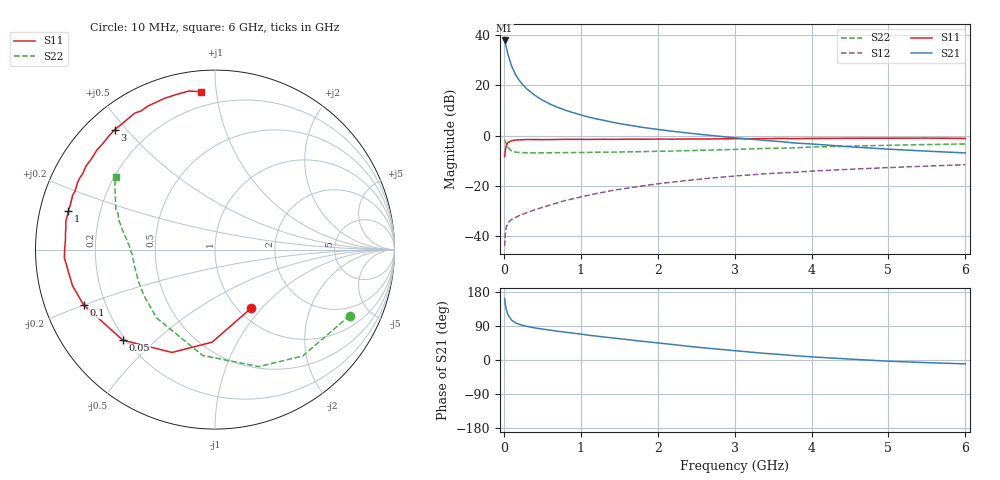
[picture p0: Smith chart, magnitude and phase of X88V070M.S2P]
! SIEMENS Small Signal Semiconductors
! BFP136W
! Si NPN RF Bipolar Junction Transistor in SOT343
! VCE = 8 V  IC = 70 mA
! Common Emitter S-Parameters:  September  1994
# GHz  S  MA  R  50
!  f  S11  S21  S12  S22
! GHz  MAG  ANG  MAG  ANG  MAG  ANG  MAG  ANG
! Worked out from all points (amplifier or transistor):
!   40 points, 10 MHz to 6 GHz, reference 50 ohm
!   highest |S21| = 37.8 dB at 10 MHz (marker M1)
!   |S21| within 3 dB of that: start of sweep to 34.34 MHz
!   unconditionally stable (mu >= 1): 640.7 MHz to 2.969 GHz
!   at 200 MHz: K = 0.58, MSG = 26.9 dB, |S12| = -31.7 dB
!   at 1.5 GHz: K = 1.11, MAG = 11.1 dB, |S12| = -21.3 dB
!   at 6 GHz: K = 0.96, MSG = 2.3 dB, |S12| = -11.5 dB
!   S11 on the Smith chart (normalised r, x): 10 MHz: 1.15, -0.88; 50 MHz: 0.19, -0.40; 100 MHz: 0.12, -0.20; 1 GHz: 0.09, +0.13; 3 GHz: 0.08, +0.46; 6 GHz: 0.11, +0.91
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0.01  0.3833 -58.2  77.81 162.0  0.0064 71.9  0.8359 -26.1
0.02  0.5161 -91.8  68.16 146.8  0.0112 60.0  0.7682 -50.5
0.03  0.6211 -112.7  58.91 135.4  0.0147 50.3  0.696 -69.5
0.05  0.7201 -135.5  43.21 120.8  0.0184 38.6  0.5938 -96.6
0.1  0.7946 -157.2  24.37 105.3  0.0217 33.7  0.5009 -130.4
0.15  0.8193 -165.8  16.65 98.3  0.0238 34.6  0.4727 -145.4
0.2  0.8248 -170.6  12.55 94.1  0.0259 36.5  0.4641 -153.7
0.25  0.8321 -174.3  10.13 91.0  0.0277 38.2  0.4609 -159.0
0.3  0.8405 -176.7  8.477 88.8  0.0296 40.4  0.4579 -162.5
0.4  0.8375 179.3  6.387 84.8  0.0337 44.6  0.4575 -167.2
0.5  0.8348 176.2  5.093 81.6  0.0376 47.8  0.458 -170.4
0.6  0.838 173.8  4.249 78.9  0.0418 50.4  0.4588 -172.5
0.8  0.8457 169.3  3.207 73.4  0.0517 54.4  0.4612 -175.3
1  0.8448 165.4  2.589 68.5  0.061 56.0  0.4642 -177.4
1.1  0.8439 162.7  2.345 65.4  0.0657 56.6  0.4661 -178.2
1.6  0.8523 153.9  1.641 54.0  0.0906 56.4  0.4773 177.9
2.2  0.8543 143.6  1.219 40.8  0.1201 53.3  0.4956 173.5
3  0.8711 129.9  0.912 24.6  0.1581 46.8  0.5344 167.0
3.2  0.8716 126.5  0.854 20.9  0.1664 45.0  0.5449 165.0
4.5  0.8884 108.5  0.602 2.4  0.2154 34.1  0.6197 153.5
5.5  0.8955 99.3  0.493 -7.0  0.2487 25.9  0.6676 146.6
6  0.8822 94.9  0.455 -10.2  0.2652 21.6  0.6855 143.6
